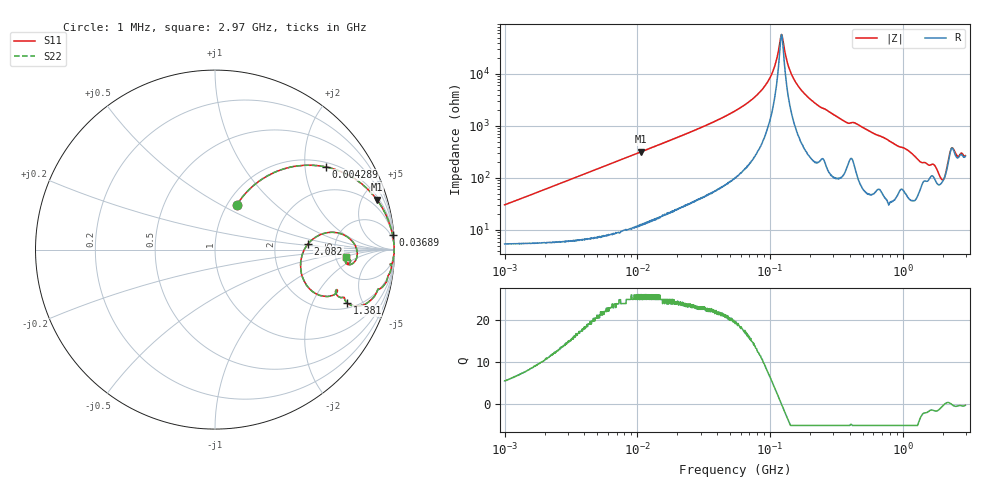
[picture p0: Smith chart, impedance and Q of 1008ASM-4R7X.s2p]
!s-Parameter Generated by FASTRON Sdn. Bhd.
!FASTRON P/N : 1008ASM-4R7X
!Keysight Technologies: E4991B_MY54100416_A.01.15
!Date: Tue Nov 21 10:15:35 2023
!Version  :Rev00  Wed Nov 22 15:09:59 2023
!Data & Calibration Information:
!Freq  S11  S21  S12  S22
!PortZ  Port1:50+j0  Port2:50+j0
!When reading reference impedance value at option line is always used.
! Remarks : This data is being provided solely for informational purposes.
# Hz S dB R 50
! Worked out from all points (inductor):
!   1599 points, 1 MHz to 2.97 GHz, reference 50 ohm
!   read as one part in series: L = 4.76 uH near 1.036 MHz
!   highest Q = 26 at 10.66 MHz (marker M1), where L = 4.77 uH
!   self-resonance near 122 MHz
!   S11 on the Smith chart (normalised r, x): 1 MHz: 1.11, +0.60; 4.289 MHz: 1.14, +2.56; 36.89 MHz: 2, +23; 1.381 GHz: 2.35, -3.75; 2.082 GHz: 3.14, +0.28; 2.97 GHz: 6.24, -1.16
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1000000  -11.10 63.9  -0.79 -15.9  -0.79 -15.9  -11.10 63.9
3804036  -2.73 39.9  -3.84 -46.8  -3.84 -46.8  -2.73 39.9
4289448  -2.28 36.8  -4.43 -50.2  -4.43 -50.2  -2.28 36.8
1.066409e7  -0.51 17.2  -10.60 -70.5  -10.60 -70.5  -0.51 17.2
1.439846e7  -0.30 13.0  -13.00 -74.8  -13.00 -74.8  -0.30 13.0
3.688738e7  -0.06 4.9  -21.40 -82.6  -21.40 -82.6  -0.06 4.9
5.477226e7  -0.03 2.9  -25.90 -84.1  -25.90 -84.1  -0.03 2.9
9.450168e7  -0.02 0.9  -36.40 -82.2  -36.40 -82.2  -0.02 0.9
1.081723e8  -0.02 0.4  -42.80 -75.6  -42.80 -75.6  -0.02 0.4
1.219755e8  -0.02 0.0  -55.20 -6.0  -55.20 -6.0  -0.02 0.0
1.368536e8  -0.02 -0.4  -43.40 74.5  -43.40 74.5  -0.02 -0.4
1.482612e8  -0.02 -0.6  -38.90 80.0  -38.90 80.0  -0.02 -0.6
2.073156e8  -0.03 -1.9  -29.70 83.9  -29.70 83.9  -0.03 -1.9
3.667557e8  -0.10 -4.6  -21.80 79.4  -21.80 79.4  -0.10 -4.6
7.846996e8  -0.25 -10.7  -14.60 76.0  -14.60 76.0  -0.25 -10.7
1.142072e9  -0.72 -17.0  -10.60 66.1  -10.60 66.1  -0.72 -17.0
1.381259e9  -2.02 -22.0  -8.01 48.1  -8.01 48.1  -2.02 -22.0
1.846379e9  -3.91 -23.6  -6.24 31.5  -6.24 31.5  -3.91 -23.6
2.081985e9  -5.68 3.5  -6.33 -3.8  -6.33 -3.8  -5.68 3.5
2.188818e9  -3.42 8.2  -9.22 -16.0  -9.22 -16.0  -3.42 8.2
2.347656e9  -2.03 -0.4  -13.60 1.7  -13.60 1.7  -2.03 -0.4
2.970126e9  -2.71 -3.4  -11.30 9.1  -11.30 9.1  -2.71 -3.4
